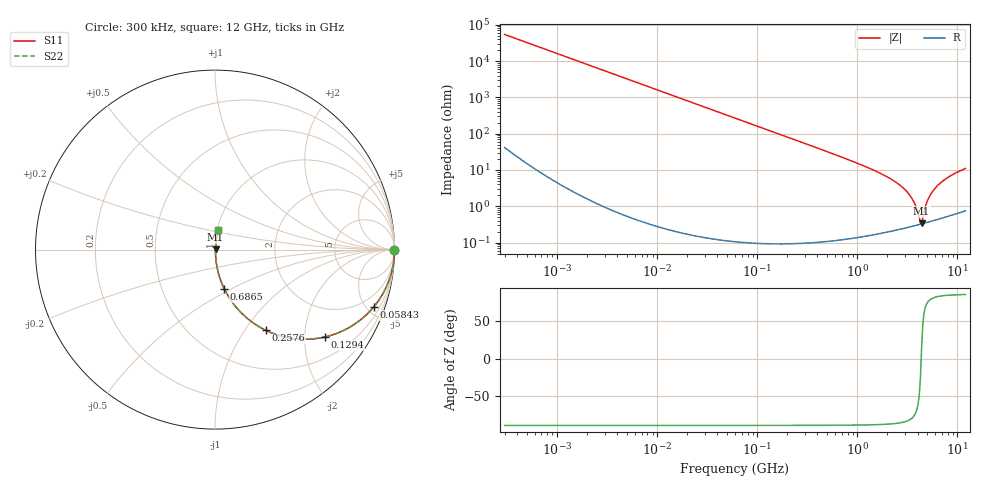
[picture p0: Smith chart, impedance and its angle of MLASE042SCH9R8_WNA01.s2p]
! MLASE042SCH9R8_WNA01  S-PARAMETER MODEL  ( General Type )
! Model Generated by TAIYO YUDEN Corporation (http://www.ty-top.com)
! Version 1.0
! TAIYO YUDEN Control No. 120810
! Copyright(c) 2012 TAIYO YUDEN CO.,LTD. All Rights Reserved.
! Product Description (link to TY-COMPAS)
! https://ds.yuden.co.jp/TYCOMPAS/or/detail?pn=MLASE042SCH9R8BWNA01&u=M
! Products Name : Multilayer Ceramic Capacitors
! Characteristics :
!  Capacitance : 9.8 pF , Rated Voltage : 16V , TCC : CH / C0H
!  Case Size : 0.4 x 0.2 / 0.016 x 0.008 [mm/inch] , Thickness : 0.2 / 0.008 [mm/inch]
!  (Conditions: Temperature = 25 degC , DC Bias Current/Voltage = 0A / 0V)
! External Node Assignments :
!  1  o---| |---o  2
! GND o---------o GND
! Frequency Range : 0.3MHz  -  12000MHz  [ 401 STEP ]
# MHz S RI R 50
! Freq[MHz].  S11 Real  S11 Imag  S21 Real  S21 Imag  S12 Real  S12 Imag  S22 Real  S22 Imag
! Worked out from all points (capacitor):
!   401 points, 300 kHz to 12 GHz, reference 50 ohm
!   read as one part in series: C = 9.79 pF near 316.3 kHz
!   lowest |Z| = 339 mohm at 4.385 GHz (marker M1)
!   series resonance near 4.344 GHz, so ESL is about 140 pH
!   S11 on the Smith chart (normalised r, x): 300 kHz: open; 58.43 MHz: 1.00, -5.56; 129.4 MHz: 1.00, -2.51; 257.6 MHz: 1.00, -1.26; 686.5 MHz: 1.00, -0.46; 12 GHz: 1.02, +0.22
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0.3  1 -0.00185  4.83e-06 0.00185  4.83e-06 0.00185  1 -0.00185
1.769972  0.9999 -0.0109  0.000121 0.0109  0.000121 0.0109  0.9999 -0.0109
10.44266  0.9959 -0.064  0.00412 0.064  0.00412 0.064  0.9959 -0.064
25.70316  0.9756 -0.1543  0.0244 0.1543  0.0244 0.1543  0.9756 -0.1543
58.43137  0.8854 -0.3184  0.1146 0.3184  0.1146 0.3184  0.8854 -0.3184
60  0.8799 -0.3249  0.1201 0.3249  0.1201 0.3249  0.8799 -0.3249
129.3602  0.6116 -0.487  0.3884 0.487  0.3884 0.487  0.6116 -0.487
257.5933  0.2835 -0.45  0.7165 0.45  0.7165 0.45  0.2835 -0.45
353.9943  0.1727 -0.3769  0.8273 0.3769  0.8273 0.3769  0.1727 -0.3769
686.4755  0.0516 -0.2187  0.9484 0.2187  0.9484 0.2187  0.0516 -0.2187
2088.533  0.00556 -0.0595  0.9944 0.0595  0.9944 0.0595  0.00556 -0.0595
2722.03  0.00367 -0.0362  0.9963 0.0362  0.9963 0.0362  0.00367 -0.0362
3276.641  0.00313 -0.0215  0.9969 0.0215  0.9969 0.0215  0.00313 -0.0215
3740.715  0.00305 -0.0114  0.9969 0.0114  0.9969 0.0114  0.00305 -0.0114
4158.869  0.00316 -0.0035  0.9968 0.0035  0.9968 0.0035  0.00316 -0.0035
4385.161  0.00328 0.000849  0.9967 -0.000849  0.9967 -0.000849  0.00328 0.000849
4502.883  0.00335 0.00343  0.9966 -0.00343  0.9966 -0.00343  0.00335 0.00343
4875.354  0.00366 0.0109  0.9963 -0.0109  0.9963 -0.0109  0.00366 0.0109
5140.631  0.00395 0.0162  0.996 -0.0162  0.996 -0.0162  0.00395 0.0162
6026.253  0.00519 0.0319  0.9948 -0.0319  0.9948 -0.0319  0.00519 0.0319
8064.993  0.00915 0.0619  0.9908 -0.0619  0.9908 -0.0619  0.00915 0.0619
12000  0.0192 0.1071  0.9808 -0.1071  0.9808 -0.1071  0.0192 0.1071
